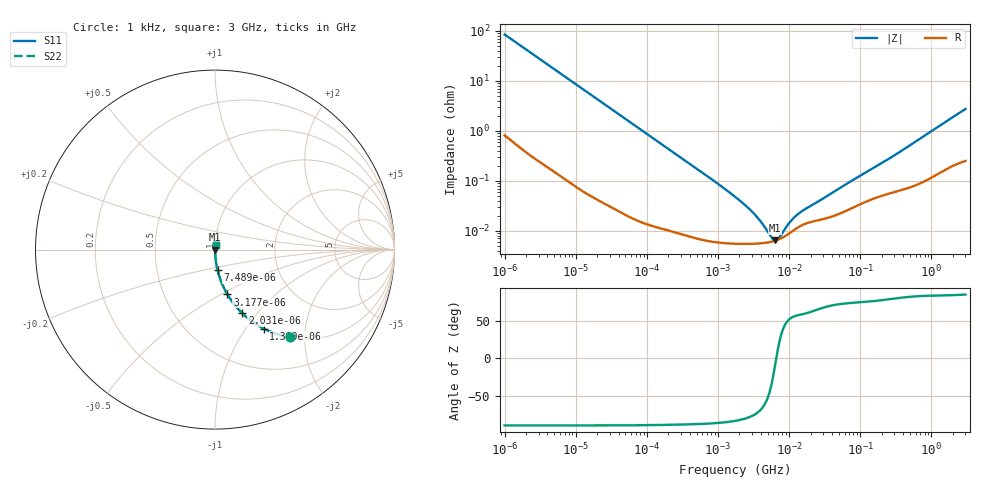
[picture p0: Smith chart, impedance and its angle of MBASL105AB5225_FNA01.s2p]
! MBASL105AB5225_FNA01  S-PARAMETER MODEL  ( Standard Model )
! Model Generated by TAIYO YUDEN Corporation (http://www.ty-top.com)
! Version 2.0
! TAIYO YUDEN Control No. 240422
! Copyright(c) 2013 TAIYO YUDEN CO.,LTD. All Rights Reserved.
! Product Description (link to TY-COMPAS)
! https://ds.yuden.co.jp/TYCOMPAS/or/detail?pn=MBASL105AB5225KFNA01&u=M
! Products Name : Multilayer Ceramic Capacitors
! Characteristics :
!  Capacitance : 2.2 [uF] , Rated Voltage : 10 [V] , TCC : X5R
!  Case Size : 1.0 x 0.5 / 0.039 x 0.02 [mm/inch] , Thickness : 0.5 / 0.02 [mm/inch]
!  (Conditions: Temperature = 25 [degC] , DC Bias Voltage = 0 [V])
! External Node Assignments :
!  1  o---| |---o  2
! GND o---------o GND
! Frequency Range : 1kHz  -  3GHz  [ 401 STEP ]
# MHZ S RI R 50
! Freq[MHz].  S11 Real  S11 Imag  S21 Real  S21 Imag  S12 Real  S12 Imag  S22 Real  S22 Imag
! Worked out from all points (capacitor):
!   401 points, 1 kHz to 3 GHz, reference 50 ohm
!   read as one part in series: C = 1.87 uF near 1.077 kHz
!   lowest |Z| = 6.38 mohm at 6.387 MHz (marker M1)
!   series resonance near 6.587 MHz, so ESL is about 310 pH
!   S11 on the Smith chart (normalised r, x): 1 kHz: 1.02, -1.70; 1.399 kHz: 1.01, -1.22; 2.031 kHz: 1.01, -0.84; 3.177 kHz: 1.00, -0.54; 7.489 kHz: 1.00, -0.23; 3 GHz: 1.00, +0.05
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0.001  0.4196 -0.4887  0.5804 0.4887  0.5804 0.4887  0.4196 -0.4887
0.001399  0.2719 -0.4404  0.7281 0.4404  0.7281 0.4404  0.2719 -0.4404
0.002031  0.1519 -0.3546  0.8481 0.3546  0.8481 0.3546  0.1519 -0.3546
0.003177  0.0693 -0.2497  0.9307 0.2497  0.9307 0.2497  0.0693 -0.2497
0.004787  0.0324 -0.1728  0.9676 0.1728  0.9676 0.1728  0.0324 -0.1728
0.007489  0.0139 -0.1129  0.9861 0.1129  0.9861 0.1129  0.0139 -0.1129
0.01216  0.0056 -0.0703  0.9944 0.0703  0.9944 0.0703  0.0056 -0.0703
0.033275  0.000956 -0.026  0.999 0.026  0.999 0.026  0.000956 -0.026
0.147855  0.000148 -0.00589  0.9999 0.00589  0.9999 0.00589  0.000148 -0.00589
0.762639  6.26e-05 -0.00114  0.9999 0.00114  0.9999 0.00114  6.26e-05 -0.00114
1.732051  5.51e-05 -0.000477  0.9999 0.000477  0.9999 0.000477  5.51e-05 -0.000477
3.03007  5.47e-05 -0.000232  0.9999 0.000232  0.9999 0.000232  5.47e-05 -0.000232
4.919932  5.79e-05 -8.04e-05  0.9999 8.04e-05  0.9999 8.04e-05  5.79e-05 -8.04e-05
5.30084  5.9e-05 -5.95e-05  0.9999 5.95e-05  0.9999 5.95e-05  5.9e-05 -5.95e-05
6.387174  6.32e-05 -8.35e-06  0.9999 8.35e-06  0.9999 8.35e-06  6.32e-05 -8.35e-06
7.696136  7.04e-05 4.21e-05  0.9999 -4.21e-05  0.9999 -4.21e-05  7.04e-05 4.21e-05
8.291982  7.44e-05 6.22e-05  0.9999 -6.22e-05  0.9999 -6.22e-05  7.44e-05 6.22e-05
12.49624  0.00011 0.000167  0.9999 -0.000167  0.9999 -0.000167  0.00011 0.000167
15.62917  0.000132 0.000217  0.9999 -0.000217  0.9999 -0.000217  0.000132 0.000217
21.06097  0.000152 0.00029  0.9998 -0.00029  0.9998 -0.00029  0.000152 0.00029
256.0921  0.000561 0.00274  0.9994 -0.00274  0.9994 -0.00274  0.000561 0.00274
3000  0.00322 0.0271  0.9968 -0.0271  0.9968 -0.0271  0.00322 0.0271
